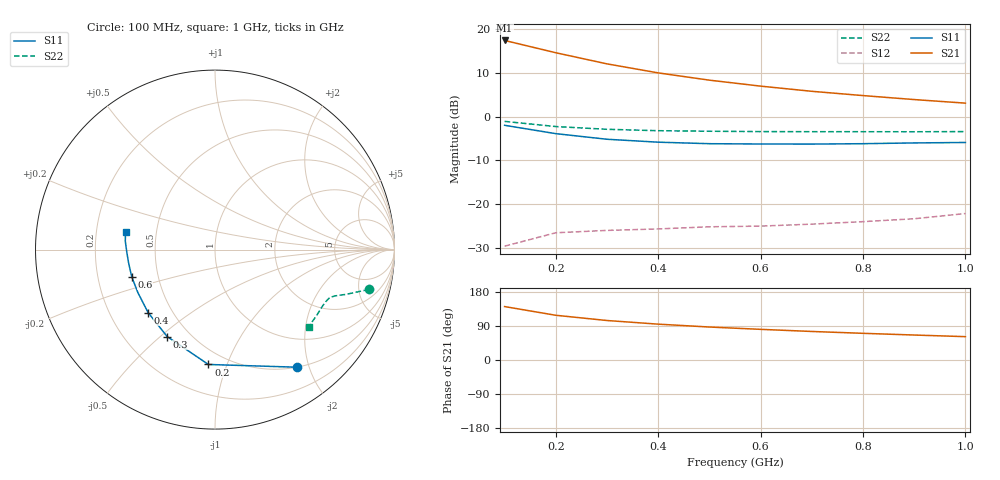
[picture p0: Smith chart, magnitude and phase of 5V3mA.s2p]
#  HZ  S  MA  R  50.0000
! Device:15GN03CA
! "! Bias:VCE=5V, IC=3mA  "
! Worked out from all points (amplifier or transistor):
!   10 points, 100 MHz to 1 GHz, reference 50 ohm
!   highest |S21| = 17.5 dB at 100 MHz (marker M1)
!   |S21| within 3 dB of that: start of sweep to 207.3 MHz
!   unconditionally stable (mu >= 1): 368.2 MHz to end of sweep
!   at 200 MHz: K = 0.56, MSG = 20.6 dB, |S12| = -26.6 dB
!   at 600 MHz: K = 1.45, MAG = 12.0 dB, |S12| = -25.0 dB
!   at 1 GHz: K = 1.51, MAG = 8.4 dB, |S12| = -22.2 dB
!   S11 on the Smith chart (normalised r, x): 100 MHz: 0.50, -1.81; 200 MHz: 0.40, -0.86; 300 MHz: 0.38, -0.53; 400 MHz: 0.37, -0.35; 600 MHz: 0.35, -0.14; 1 GHz: 0.33, +0.09
1e8  0.799 -55.1  7.483 141.0  0.033 59.9  0.886 -14.5
2e8  0.641 -93.3  5.412 118.0  0.047 44.3  0.773 -18.8
3e8  0.553 -118.8  4.036 104.2  0.05 40.2  0.719 -21.0
4e8  0.512 -136.7  3.182 94.6  0.052 40.7  0.693 -22.6
5e8  0.492 -150.9  2.627 87.0  0.055 44.7  0.683 -24.9
6e8  0.488 -162.0  2.244 80.9  0.056 49.3  0.677 -27.4
7e8  0.487 -171.1  1.958 75.3  0.059 55.4  0.675 -30.2
8e8  0.492 -178.7  1.749 70.4  0.063 62.4  0.675 -33.3
9e8  0.502 174.6  1.575 65.9  0.068 67.8  0.674 -36.4
1e9  0.508 168.9  1.433 61.6  0.078 74.1  0.677 -39.3
